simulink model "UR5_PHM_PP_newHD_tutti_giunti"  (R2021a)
settings: Solver=ode14x  StartTime=0.0  StopTime=Sim.time  FixedStep=Sim.dt  MaxStep=Sim.dt  RelTol=1e-3  EnableMultiTasking=on
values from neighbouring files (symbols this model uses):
  alpha_n = 0.98*pi/180    (= 0.0171042266695)    [parameters.m]
  alpha_t = 30*pi/180    (= 0.523598775598)    [parameters.m]
  alpha_TTS = 0    [parameters.m]
  alpha_Tw_L = -6.9e-4    (= -0.00069)    [parameters.m]
  alpha_Tw_R = 3.9e-3    (= 0.0039)    [parameters.m]
  Beta_TTS = 0    [parameters.m]
  c1 = 1e-2    (= 0.01)    [parameters.m]
  c2 = 1e-2    (= 0.01)    [parameters.m]
  c3 = 1e-2    (= 0.01)    [parameters.m]
  c4 = 1e-2    (= 0.01)    [parameters.m]
  c5 = 1e-2    (= 0.01)    [parameters.m]
  c6 = 1e-2    (= 0.01)    [parameters.m]
  Cb1 = 1.8e3    (= 1800)    [parameters.m]
  Cb2 = 1.8e3    (= 1800)    [parameters.m]
  Cb3 = 1.8e3    (= 1800)    [parameters.m]
  Cb4 = 1.8e3    (= 1800)    [parameters.m]
  Cb5 = 1.8e3    (= 1800)    [parameters.m]
  Cb6 = 1.8e3    (= 1800)    [parameters.m]
  Cth_housing = 153.90    (= 153.9)    [parameters.m]
  Cth_w = 74.20    (= 74.2)    [parameters.m]
  dt_PP = 0.05    [parameters.m]
  Fric1 = [fc_1/2 1e1 fc_1 fv_1]    [parameters.m]
  Fric2 = [fc_2/2 1e1 fc_2 fv_2]    [parameters.m]
  Fric3 = [fc_3/2 1e1 fc_3 fv_3]    [parameters.m]
  Fric4 = [fc_4/2 1e1 fc_4 fv_4]    [parameters.m]
  Fric5 = [fc_5/2 1e1 fc_5 fv_5]    [parameters.m]
  Fric6 = [fc_6/2 1e1 fc_6 fv_6]    [parameters.m]
  Hth_housing = 0.30    (= 0.3)    [parameters.m]
  Hth_w = 1.14    [parameters.m]
  I_actual = I_actual(1:10,:)    [trajcutting.m]
  J_CS1 = 7.12e-5    (= 7.12e-05)    [parameters.m]
  J_CS2 = 7.12e-5    (= 7.12e-05)    [parameters.m]
  J_CS3 = 7.12e-5    (= 7.12e-05)    [parameters.m]
  J_CS4 = 6e-6    (= 6e-06)    [parameters.m]
  J_CS5 = 6e-6    (= 6e-06)    [parameters.m]
  J_CS6 = 6e-6    (= 6e-06)    [parameters.m]
  J_FS1 = 1.62e-7    (= 1.62e-07)    [parameters.m]
  J_FS2 = 1.62e-7    (= 1.62e-07)    [parameters.m]
  J_FS3 = 1.62e-7    (= 1.62e-07)    [parameters.m]
  J_FS4 = 4.97e-8    (= 4.97e-08)    [parameters.m]
  J_FS5 = 4.97e-8    (= 4.97e-08)    [parameters.m]
  J_FS6 = 4.97e-8    (= 4.97e-08)    [parameters.m]
  J_WG1 = 3.56e-5    (= 3.56e-05)    [parameters.m]
  J_WG2 = 3.56e-5    (= 3.56e-05)    [parameters.m]
  J_WG3 = 3.56e-5    (= 3.56e-05)    [parameters.m]
  J_WG4 = 3e-6    (= 3e-06)    [parameters.m]
  J_WG5 = 3e-6    (= 3e-06)    [parameters.m]
  J_WG6 = 3e-6    (= 3e-06)    [parameters.m]
  K_i = 1    [parameters.m]
  K_p = 1    [parameters.m]
  K_torsCS1 = 4.78e6    (= 4780000)    [parameters.m]
  K_torsCS2 = 4.78e6    (= 4780000)    [parameters.m]
  K_torsCS3 = 4.78e6    (= 4780000)    [parameters.m]
  K_torsCS4 = 1.06e6    (= 1060000)    [parameters.m]
  K_torsCS5 = 1.06e6    (= 1060000)    [parameters.m]
  K_torsCS6 = 1.06e6    (= 1060000)    [parameters.m]
  K_torsWG1 = 9.56e5    (= 956000)    [parameters.m]
  K_torsWG2 = 9.56e5    (= 956000)    [parameters.m]
  K_torsWG3 = 9.56e5    (= 956000)    [parameters.m]
  K_torsWG4 = 1.84e5    (= 184000)    [parameters.m]
  K_torsWG5 = 1.84e5    (= 184000)    [parameters.m]
  K_torsWG6 = 1.84e5    (= 184000)    [parameters.m]
  K_v = 1    [parameters.m]
  Kb1 = 0.51e8    (= 51000000)    [parameters.m]
  Kb2 = 0.51e8    (= 51000000)    [parameters.m]
  Kb3 = 0.51e8    (= 51000000)    [parameters.m]
  Kb4 = 1.98e7    (= 19800000)    [parameters.m]
  Kb5 = 1.98e7    (= 19800000)    [parameters.m]
  Kb6 = 1.98e7    (= 19800000)    [parameters.m]
  Km1 = 1.2e9    (= 1200000000)    [parameters.m]
  Km2 = 1.2e9    (= 1200000000)    [parameters.m]
  Km3 = 1.2e9    (= 1200000000)    [parameters.m]
  Km4 = 5.55e8    (= 555000000)    [parameters.m]
  Km5 = 5.55e8    (= 555000000)    [parameters.m]
  Km6 = 5.55e8    (= 555000000)    [parameters.m]
  Kt1 = 0.96e5    (= 96000)    [parameters.m]
  Kt2 = 0.96e5    (= 96000)    [parameters.m]
  Kt3 = 0.96e5    (= 96000)    [parameters.m]
  Kt4 = 1.15e4    (= 11500)    [parameters.m]
  Kt5 = 1.15e4    (= 11500)    [parameters.m]
  Kt6 = 1.15e4    (= 11500)    [parameters.m]
  L = Motor.L_2/2    [parameters.m]
  m2 = polyfit(Temp(:,2),pBn_UR5_f_Temp(:,2),1)    [parameters.m]
  mb2 = polyfit(Temp(:,8),pBn_UR5_f_Temp(:,8),1)    [parameters.m]
  pickTime = t_pick(traj)    [parameters.m]
  placeTime = t_place(traj)    [parameters.m]
  q0 = q_target(1,:)    [testlaw_PP.m]
  q_CS01 = x(6)    [parameters.m]
  q_CS02 = x(6)    [parameters.m]
  q_CS03 = x(6)    [parameters.m]
  q_CS04 = x(6)    [parameters.m]
  q_CS05 = x(6)    [parameters.m]
  q_CS06 = x(6)    [parameters.m]
  q_WG01 = x(1)    [parameters.m]
  q_WG02 = x(1)    [parameters.m]
  q_WG03 = x(1)    [parameters.m]
  q_WG04 = x(1)    [parameters.m]
  q_WG05 = x(1)    [parameters.m]
  q_WG06 = x(1)    [parameters.m]
  quant_i = [Motor.imax1 Motor.imax2      Motor.imax3 Motor.imax4 Motor.imax5 Motor.imax6]/2^16    [parameters.m]
  R = Motor.R_2/2    [parameters.m]
  rg1 = 0.028    [parameters.m]
  rg2 = 0.028    [parameters.m]
  rg3 = 0.028    [parameters.m]
  rg4 = 0.0155    [parameters.m]
  rg5 = 0.0155    [parameters.m]
  rg6 = 0.0155    [parameters.m]
  sigma_p = 444.29    [parameters.m]
  sigma_v = 2*pi*1000    (= 6283.18530718)    [parameters.m]
  stiff_red = 1    [parameters.m]
  T_0 = Sim.temp    [parameters.m]
  T_switch = 1e-4    (= 0.0001)    [parameters.m]
  tau_i = 1/(fc_i*2*pi)    (= 7.95774715459e-05)    [parameters.m]
  U_s = 48    [parameters.m]
  var_i = 1e-1*[.0167 .0184 .0144 .0016      .0011 .0007]    [parameters.m]
  var_p = 1e-6*[.0943 .3877      .3478 .5436 .3400 .2081]    [parameters.m]
  var_v = 1e-4*[.0738 .1452      .1564 .4623 .1824 .0917]    [parameters.m]
  Wf_TTS_0 = 0    [parameters.m]
  Wf_TTS_ONOFF = 0    [parameters.m]
  x2_01 = x(3)    [parameters.m]
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undefined symbols (not defined in the file or in its folder): deg, Driver1, Driver2, Driver3, Driver4, Driver5, Driver6, elseif, geom, Ground, J1, J2, J3, J4, J5, J6, kg, L1, L2, L3, L4, L5, L6, LINK0, LINK1, LINK2, LINK3, LINK4, LINK5, LINK6, m, Motor, N, payload, ROBOTIQ_FT, s, Sim, Tool, X, Y, Z
libraries: sm_lib x35, nesl_utility x30, simulink x23, simulink_extras x11, spsTriangleGeneratorLib x6
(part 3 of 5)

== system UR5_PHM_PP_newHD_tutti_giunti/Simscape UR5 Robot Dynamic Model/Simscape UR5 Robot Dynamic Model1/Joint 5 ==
  T5 : Inport
  A_45*E_1 : sm_lib/Frames and Transforms/Rigid Transform  TranslationMethod=Cartesian  TranslationStandardOffset=0  TranslationLengthUnit=mm  TranslationStandardAxis=+Z  TranslationCartesianOffset=A45t  TranslationROffset=0  TranslationROffsetUnits=m  TranslationZOffset=0  TranslationZOffsetUnits=m  TranslationThetaOffset=0  TranslationThetaOffsetUnits=deg  RotationMethod=None  RotationAngleUnits=deg  RotationStandardAxis=+Z  RotationAngle=0.0  RotationArbitraryAxis=[0 0 1]  FollAlignAxisA=+X  BaseAlignAxisA=+Y  FollAlignAxisB=+Y  BaseAlignAxisB=+Z  RotationSequenceAxes=FollowerAxes  RotationSequence=XYX  RotationSequenceAngles=[0 0 0]  RotationSequenceAnglesUnits=deg  RotationMatrix=A45r
  A_45*E_45 : sm_lib/Frames and Transforms/Rigid Transform  TranslationMethod=None  TranslationStandardOffset=0  TranslationLengthUnit=mm  TranslationStandardAxis=+Z  TranslationCartesianOffset=A45t  TranslationROffset=0  TranslationROffsetUnits=m  TranslationZOffset=0  TranslationZOffsetUnits=m  TranslationThetaOffset=0  TranslationThetaOffsetUnits=deg  RotationMethod=RotationMatrix  RotationAngleUnits=deg  RotationStandardAxis=+Z  RotationAngle=0.0  RotationArbitraryAxis=[0 0 1]  FollAlignAxisA=+X  BaseAlignAxisA=+Y  FollAlignAxisB=+Y  BaseAlignAxisB=+Z  RotationSequenceAxes=FollowerAxes  RotationSequence=XYX  RotationSequenceAngles=[0 0 0]  RotationSequenceAnglesUnits=deg  RotationMatrix=A45r
  Mux : Mux  Inputs=3
  PS-Simulink Converter1 : nesl_utility/PS-Simulink Converter  PhysicalDomain=network_engine_domain  SubClassName=ps_output  LeftPortType=input  RightPortType=output  PseudoPeriodic=off  Frequencies=[]  Unit=1  AffineConversion=off
  PS-Simulink Converter2 : nesl_utility/PS-Simulink Converter  PhysicalDomain=network_engine_domain  SubClassName=ps_output  LeftPortType=input  RightPortType=output  PseudoPeriodic=off  Frequencies=[]  Unit=1  AffineConversion=off
  PS-Simulink Converter7 : nesl_utility/PS-Simulink Converter  PhysicalDomain=network_engine_domain  SubClassName=ps_output  LeftPortType=input  RightPortType=output  PseudoPeriodic=off  Frequencies=[]  Unit=1  AffineConversion=off
  Revolute Joint5 : sm_lib/Joints/Revolute Joint  JointMode=Normal  SenseConstraintForce=off  SenseConstraintForceX=off  SenseConstraintForceY=off  SenseConstraintForceZ=off  SenseConstraintTorque=off  SenseConstraintTorqueX=off  SenseConstraintTorqueY=off  SenseConstraintTorqueZ=off  SenseTotalForce=off  SenseTotalForceX=off  SenseTotalForceY=off  SenseTotalForceZ=off  SenseTotalTorque=off  SenseTotalTorqueX=off  SenseTotalTorqueY=off  SenseTotalTorqueZ=off  CompositeWrenchDir=FollowerOnBase  CompositeWrenchFrame=BaseFrame  EquilibriumPosition=0  EquilibriumPositionUnits=deg  SpringStiffness=0  SpringStiffnessUnits=N*m/deg  DampingCoefficient=0  DampingCoefficientUnits=N*m/(deg/s)  TorqueActuationMode=InputTorque  MotionActuationMode=ComputedMotion  SensePosition=on  SenseVelocity=on  SenseAcceleration=on  SenseTorqueForce=off  SenseLowerLimitTorqueForce=off  SenseUpperLimitTorqueForce=off  LowerLimitSpecify=on  LowerLimitBound=-J5.al  LowerLimitBoundUnits=deg  LowerLimitStiffness=1e4  LowerLimitStiffnessUnits=N*m/deg  LowerLimitDamping=10  LowerLimitDampingUnits=N*m/(deg/s)  LowerLimitTransitionRegionWidth=0.1  LowerLimitTransitionRegionWidthUnits=deg  UpperLimitSpecify=on  UpperLimitBound=J5.al  UpperLimitBoundUnits=deg  UpperLimitStiffness=1e4  UpperLimitStiffnessUnits=N*m/deg  UpperLimitDamping=10  UpperLimitDampingUnits=N*m/(deg/s)  UpperLimitTransitionRegionWidth=0.1  UpperLimitTransitionRegionWidthUnits=deg  PositionTargetSpecify=on  PositionTargetPriority=Low  PositionTargetValue=q0(5)  PositionTargetValueUnits=rad  VelocityTargetSpecify=off  VelocityTargetPriority=High  VelocityTargetValue=0  VelocityTargetValueUnits=deg/s
  Simulink-PS Converter : nesl_utility/Simulink-PS Converter  PhysicalDomain=network_engine_domain  SubClassName=ps_input  LeftPortType=input  RightPortType=output  PseudoPeriodic=off  Frequencies=[]  NoiseDistribution=none  NoiseParameters=[]  Unit=1  AffineConversion=off  FilteringAndDerivatives=provide  SimscapeFilterOrder=1  InputFilterTimeConstant=0.001  UdotUserProvided=0
  Link 4 : PMIOPort  Side=Left
  Link 5 : PMIOPort  Port=2  Side=Right
  q5,qd5,qdd5 : Outport
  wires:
  PS-Simulink Converter1/1 -> Mux/1
  T5/1 -> Simulink-PS Converter/1
  Mux/1 -> q5,qd5,qdd5/1
  PS-Simulink Converter7/1 -> Mux/2
  PS-Simulink Converter2/1 -> Mux/3
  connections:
  A_45*E_45/RConn1 -- A_45*E_1/LConn1
  A_45*E_1/RConn1 -- Revolute Joint5/LConn1
  A_45*E_45/LConn1 -- Link 4/RConn1
  Revolute Joint5/RConn1 -- Link 5/RConn1
  Revolute Joint5/RConn4 -- PS-Simulink Converter2/LConn1
  Revolute Joint5/LConn2 -- Simulink-PS Converter/RConn1
  Revolute Joint5/RConn3 -- PS-Simulink Converter7/LConn1
  Revolute Joint5/RConn2 -- PS-Simulink Converter1/LConn1

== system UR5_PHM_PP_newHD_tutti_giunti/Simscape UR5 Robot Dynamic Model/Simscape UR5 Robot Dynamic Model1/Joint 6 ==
  T6 : Inport
  A_56*E_1 : sm_lib/Frames and Transforms/Rigid Transform  TranslationMethod=Cartesian  TranslationStandardOffset=0  TranslationLengthUnit=mm  TranslationStandardAxis=+Z  TranslationCartesianOffset=A56t  TranslationROffset=0  TranslationROffsetUnits=m  TranslationZOffset=0  TranslationZOffsetUnits=m  TranslationThetaOffset=0  TranslationThetaOffsetUnits=deg  RotationMethod=None  RotationAngleUnits=deg  RotationStandardAxis=+Z  RotationAngle=0.0  RotationArbitraryAxis=[0 0 1]  FollAlignAxisA=+X  BaseAlignAxisA=+Y  FollAlignAxisB=+Y  BaseAlignAxisB=+Z  RotationSequenceAxes=FollowerAxes  RotationSequence=XYX  RotationSequenceAngles=[0 0 0]  RotationSequenceAnglesUnits=deg  RotationMatrix=A56r
  A_56*E_56 : sm_lib/Frames and Transforms/Rigid Transform  TranslationMethod=None  TranslationStandardOffset=0  TranslationLengthUnit=mm  TranslationStandardAxis=+Z  TranslationCartesianOffset=A56t  TranslationROffset=0  TranslationROffsetUnits=m  TranslationZOffset=0  TranslationZOffsetUnits=m  TranslationThetaOffset=0  TranslationThetaOffsetUnits=deg  RotationMethod=RotationMatrix  RotationAngleUnits=deg  RotationStandardAxis=+Z  RotationAngle=0.0  RotationArbitraryAxis=[0 0 1]  FollAlignAxisA=+X  BaseAlignAxisA=+Y  FollAlignAxisB=+Y  BaseAlignAxisB=+Z  RotationSequenceAxes=FollowerAxes  RotationSequence=XYX  RotationSequenceAngles=[0 0 0]  RotationSequenceAnglesUnits=deg  RotationMatrix=A56r
  Mux : Mux  Inputs=3
  PS-Simulink Converter1 : nesl_utility/PS-Simulink Converter  PhysicalDomain=network_engine_domain  SubClassName=ps_output  LeftPortType=input  RightPortType=output  PseudoPeriodic=off  Frequencies=[]  Unit=1  AffineConversion=off
  PS-Simulink Converter2 : nesl_utility/PS-Simulink Converter  PhysicalDomain=network_engine_domain  SubClassName=ps_output  LeftPortType=input  RightPortType=output  PseudoPeriodic=off  Frequencies=[]  Unit=1  AffineConversion=off
  PS-Simulink Converter7 : nesl_utility/PS-Simulink Converter  PhysicalDomain=network_engine_domain  SubClassName=ps_output  LeftPortType=input  RightPortType=output  PseudoPeriodic=off  Frequencies=[]  Unit=1  AffineConversion=off
  Revolute Joint6 : sm_lib/Joints/Revolute Joint  JointMode=Normal  SenseConstraintForce=off  SenseConstraintForceX=off  SenseConstraintForceY=off  SenseConstraintForceZ=off  SenseConstraintTorque=off  SenseConstraintTorqueX=off  SenseConstraintTorqueY=off  SenseConstraintTorqueZ=off  SenseTotalForce=off  SenseTotalForceX=off  SenseTotalForceY=off  SenseTotalForceZ=off  SenseTotalTorque=off  SenseTotalTorqueX=off  SenseTotalTorqueY=off  SenseTotalTorqueZ=off  CompositeWrenchDir=FollowerOnBase  CompositeWrenchFrame=BaseFrame  EquilibriumPosition=0  EquilibriumPositionUnits=deg  SpringStiffness=0  SpringStiffnessUnits=N*m/deg  DampingCoefficient=0  DampingCoefficientUnits=N*m/(deg/s)  TorqueActuationMode=InputTorque  MotionActuationMode=ComputedMotion  SensePosition=on  SenseVelocity=on  SenseAcceleration=on  SenseTorqueForce=off  SenseLowerLimitTorqueForce=off  SenseUpperLimitTorqueForce=off  LowerLimitSpecify=on  LowerLimitBound=-J6.al  LowerLimitBoundUnits=deg  LowerLimitStiffness=1e4  LowerLimitStiffnessUnits=N*m/deg  LowerLimitDamping=10  LowerLimitDampingUnits=N*m/(deg/s)  LowerLimitTransitionRegionWidth=0.1  LowerLimitTransitionRegionWidthUnits=deg  UpperLimitSpecify=on  UpperLimitBound=J6.al  UpperLimitBoundUnits=deg  UpperLimitStiffness=1e4  UpperLimitStiffnessUnits=N*m/deg  UpperLimitDamping=10  UpperLimitDampingUnits=N*m/(deg/s)  UpperLimitTransitionRegionWidth=0.1  UpperLimitTransitionRegionWidthUnits=deg  PositionTargetSpecify=on  PositionTargetPriority=Low  PositionTargetValue=q0(6)  PositionTargetValueUnits=rad  VelocityTargetSpecify=off  VelocityTargetPriority=High  VelocityTargetValue=0  VelocityTargetValueUnits=deg/s
  Simulink-PS Converter : nesl_utility/Simulink-PS Converter  PhysicalDomain=network_engine_domain  SubClassName=ps_input  LeftPortType=input  RightPortType=output  PseudoPeriodic=off  Frequencies=[]  NoiseDistribution=none  NoiseParameters=[]  Unit=1  AffineConversion=off  FilteringAndDerivatives=provide  SimscapeFilterOrder=1  InputFilterTimeConstant=0.001  UdotUserProvided=0
  Link 5 : PMIOPort  Side=Left
  Link 6 : PMIOPort  Port=2  Side=Right
  q6,qd6,qdd6 : Outport
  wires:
  PS-Simulink Converter1/1 -> Mux/1
  T6/1 -> Simulink-PS Converter/1
  Mux/1 -> q6,qd6,qdd6/1
  PS-Simulink Converter7/1 -> Mux/2
  PS-Simulink Converter2/1 -> Mux/3
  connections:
  A_56*E_1/LConn1 -- A_56*E_56/RConn1
  Revolute Joint6/LConn1 -- A_56*E_1/RConn1
  Revolute Joint6/RConn1 -- Link 6/RConn1
  A_56*E_56/LConn1 -- Link 5/RConn1
  Revolute Joint6/RConn4 -- PS-Simulink Converter2/LConn1
  Revolute Joint6/LConn2 -- Simulink-PS Converter/RConn1
  Revolute Joint6/RConn3 -- PS-Simulink Converter7/LConn1
  Revolute Joint6/RConn2 -- PS-Simulink Converter1/LConn1

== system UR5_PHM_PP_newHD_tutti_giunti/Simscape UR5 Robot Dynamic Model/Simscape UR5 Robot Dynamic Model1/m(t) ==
  Add : Sum  Inputs=++++
  Ramp : simulink/Sources/Ramp  slope=payload.m/dt_PP  start=pickTime  InitialOutput=0.001
  Ramp1 : simulink/Sources/Ramp  slope=-payload.m/dt_PP  start=pickTime+dt_PP  InitialOutput=0.001
  Ramp2 : simulink/Sources/Ramp  slope=-payload.m/dt_PP  start=placeTime  InitialOutput=0.001
  Ramp3 : simulink/Sources/Ramp  slope=payload.m/dt_PP  start=placeTime+dt_PP  InitialOutput=0.001
  Out1 : Outport
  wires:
  Ramp2/1 -> Add/3
  Ramp/1 -> Add/1
  Ramp3/1 -> Add/4
  Ramp1/1 -> Add/2
  Add/1 -> Out1/1

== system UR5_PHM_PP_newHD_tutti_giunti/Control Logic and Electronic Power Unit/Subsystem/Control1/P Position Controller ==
  q_error : Inport
  "[-pi*tau,pi*tau]" : Saturate  UpperLimit=pi*Motor.tau  LowerLimit=-pi*Motor.tau
  kp_p : Gain  Gain=Driver1.Pp
  qdm_ref : Outport
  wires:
  kp_p/1 -> "[-pi*tau,pi*tau]"/1
  q_error/1 -> kp_p/1
  "[-pi*tau,pi*tau]"/1 -> qdm_ref/1

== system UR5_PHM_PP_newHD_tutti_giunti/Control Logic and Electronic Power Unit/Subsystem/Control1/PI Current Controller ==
  i_error : Inport
  Integral Contribution : Scope
  Integrator : Integrator
  Proportional Contribution : Scope
  Sum3 : Sum  Inputs=|++
  "[-U_s,U_s]" : Saturate  UpperLimit=U_s  LowerLimit=-U_s
  ki_i : Gain  Gain=Driver1.Ii
  kp_i : Gain  Gain=Driver1.Pi
  V_ref : Outport
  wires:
  i_error/1 -> ki_i/1, kp_i/1
  kp_i/1 -> Sum3/1, Proportional Contribution/1
  "[-U_s,U_s]"/1 -> V_ref/1
  Sum3/1 -> "[-U_s,U_s]"/1
  ki_i/1 -> Integrator/1
  Integrator/1 -> Integral Contribution/1, Sum3/2

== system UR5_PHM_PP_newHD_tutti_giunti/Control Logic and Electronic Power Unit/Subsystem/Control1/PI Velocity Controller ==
  qdm_error : Inport
  Current : Scope
  Integral Contribution : Scope
  Integrator : Integrator
  Proportional Contribution : Scope
  Sum3 : Sum  Inputs=|++
  "[-i_max,i_max]" : Saturate  UpperLimit=Motor.imax1  LowerLimit=-Motor.imax1
  ki_v : Gain  Gain=Driver1.Iv
  kp_v : Gain  Gain=Driver1.Pv
  i_ref : Outport
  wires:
  Sum3/1 -> "[-i_max,i_max]"/1
  "[-i_max,i_max]"/1 -> Current/1, i_ref/1
  kp_v/1 -> Proportional Contribution/1, Sum3/1
  qdm_error/1 -> ki_v/1, kp_v/1
  ki_v/1 -> Integrator/1
  Integrator/1 -> Sum3/2, Integral Contribution/1

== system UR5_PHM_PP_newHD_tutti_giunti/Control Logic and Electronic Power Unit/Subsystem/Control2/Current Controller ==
  i_ref : Inport
  i_FB [dq0] : Inport  Port=2
  Controller - d : Subsystem
  Controller - q : Subsystem
  Demux : Demux  Outputs=3
  Mux : Mux  Inputs=3
  V[d,q,0] : Outport
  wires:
  Controller - d/1(v*d) -> Mux/1  "vd_j2"
  Demux/3 -> Mux/3  "i0_j2"
  Controller - q/1(v*q) -> Mux/2  "vq_j2"
  Demux/2 -> Controller - q/2(Iq)  "iq_j2"
  i_ref/1 -> Controller - q/1(i*)
  i_FB [dq0]/1 -> Demux/1
  Demux/1 -> Controller - d/1(id)  "id_j2"
  Mux/1 -> V[d,q,0]/1

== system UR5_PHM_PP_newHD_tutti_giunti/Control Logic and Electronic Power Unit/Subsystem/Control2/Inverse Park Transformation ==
  V[d,q,0] : Inport
  qm : Inport  Port=2
  A11 : Fcn  Expr=sin(u(1))
  A12 : Fcn  Expr=cos(u(1))
  A13 : Fcn  Expr=sqrt(2)/2
  A21 : Fcn  Expr=sin(u(1)-2/3*pi)
  A22 : Fcn  Expr=cos(u(1)-2/3*pi)
  A23 : Fcn  Expr=sqrt(2)/2
  A31 : Fcn  Expr=sin(u(1)+2/3*pi)
  A32 : Fcn  Expr=cos(u(1)+2/3*pi)
  A33 : Fcn  Expr=sqrt(2)/2
  Gain : Gain  Gain=sqrt(2/3)
  Gain1 : Gain  Gain=Motor.Zp_2
  Matrix : Subsystem
  Product : Product  Multiplication=Matrix(*)  RndMeth=Zero
  V[a,b,c] : Outport  VectorParamsAs1DForOutWhenUnconnected=off
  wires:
  Product/1 -> V[a,b,c]/1
  V[d,q,0]/1 -> Product/2
  Gain/1 -> Product/1
  Gain1/1 -> A22/1, A21/1, A11/1, A12/1, A13/1, A31/1, A32/1, A33/1, A23/1
  A11/1 -> Matrix/1(A11)
  A23/1 -> Matrix/6(A23)
  A12/1 -> Matrix/2(A12)
  A21/1 -> Matrix/4(A21)
  qm/1 -> Gain1/1
  A33/1 -> Matrix/9(A33)
  Matrix/1(Out1) -> Gain/1
  A13/1 -> Matrix/3(A13)
  A22/1 -> Matrix/5(A22)
  A32/1 -> Matrix/8(A32)
  A31/1 -> Matrix/7(A31)

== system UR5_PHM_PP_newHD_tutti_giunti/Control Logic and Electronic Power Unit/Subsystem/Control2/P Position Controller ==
  q_error : Inport
  "[-pi*tau,pi*tau]" : Saturate  UpperLimit=pi*Motor.tau  LowerLimit=-pi*Motor.tau
  kp_p : Gain  Gain=Driver2.Pp
  qdm_ref : Outport
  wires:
  q_error/1 -> kp_p/1
  "[-pi*tau,pi*tau]"/1 -> qdm_ref/1
  kp_p/1 -> "[-pi*tau,pi*tau]"/1

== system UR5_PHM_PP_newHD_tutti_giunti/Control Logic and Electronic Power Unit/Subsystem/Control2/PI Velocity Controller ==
  qdm_error : Inport
  Add : Sum
  Integral Contribution : Scope
  Integrator1 : Integrator
  Proportional Contribution : Scope
  Scope i_ref : Scope  NumInputPorts=2
  "[-i_max,i_max]" : Saturate  UpperLimit=Motor.imax2  LowerLimit=-Motor.imax2
  ki_v : Gain  Gain=Driver2.Iv
  kp_v : Gain  Gain=Driver2.Pv
  i_ref : Outport
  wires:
  Integrator1/1 -> Integral Contribution/1, Add/2
  qdm_error/1 -> ki_v/1, kp_v/1
  kp_v/1 -> Proportional Contribution/1, Add/1
  Add/1 -> Scope i_ref/1, "[-i_max,i_max]"/1
  "[-i_max,i_max]"/1 -> i_ref/1, Scope i_ref/2
  ki_v/1 -> Integrator1/1

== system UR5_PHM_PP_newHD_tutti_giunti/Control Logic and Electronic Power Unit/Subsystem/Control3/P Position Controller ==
  q_error : Inport
  "[-pi*tau,pi*tau]" : Saturate  UpperLimit=pi*Motor.tau  LowerLimit=-pi*Motor.tau
  kp_p : Gain  Gain=Driver2.Pp
  qdm_ref : Outport
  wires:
  kp_p/1 -> "[-pi*tau,pi*tau]"/1
  q_error/1 -> kp_p/1
  "[-pi*tau,pi*tau]"/1 -> qdm_ref/1

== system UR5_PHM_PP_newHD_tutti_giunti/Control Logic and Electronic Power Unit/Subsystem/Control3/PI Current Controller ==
  i_error : Inport
  Integral Contribution : Scope
  Integrator : Integrator
  Proportional Contribution : Scope
  Sum3 : Sum  Inputs=|++
  "[-U_s,U_s]" : Saturate  UpperLimit=U_s  LowerLimit=-U_s
  ki_i : Gain  Gain=Driver3.Ii
  kp_i : Gain  Gain=Driver3.Pi
  V_ref : Outport
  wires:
  i_error/1 -> ki_i/1, kp_i/1
  kp_i/1 -> Sum3/1, Proportional Contribution/1
  "[-U_s,U_s]"/1 -> V_ref/1
  Sum3/1 -> "[-U_s,U_s]"/1
  Integrator/1 -> Sum3/2, Integral Contribution/1
  ki_i/1 -> Integrator/1

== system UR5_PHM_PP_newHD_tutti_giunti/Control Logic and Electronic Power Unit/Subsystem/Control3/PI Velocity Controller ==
  qdm_error : Inport
  Integral Contribution : Scope
  Integrator : Integrator
  Proportional Contribution : Scope
  Sum3 : Sum  Inputs=|++
  "[-i_max,i_max]" : Saturate  UpperLimit=Motor.imax3  LowerLimit=-Motor.imax3
  ki_v : Gain  Gain=Driver3.Iv
  kp_v : Gain  Gain=Driver3.Pv
  i_ref : Outport
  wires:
  Sum3/1 -> "[-i_max,i_max]"/1
  "[-i_max,i_max]"/1 -> i_ref/1
  kp_v/1 -> Proportional Contribution/1, Sum3/1
  qdm_error/1 -> ki_v/1, kp_v/1
  ki_v/1 -> Integrator/1
  Integrator/1 -> Sum3/2, Integral Contribution/1

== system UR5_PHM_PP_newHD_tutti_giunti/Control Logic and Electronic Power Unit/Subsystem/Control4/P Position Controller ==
  q_error : Inport
  "[-pi*tau,pi*tau]" : Saturate  UpperLimit=pi*Motor.tau  LowerLimit=-pi*Motor.tau
  kp_p : Gain  Gain=Driver4.Pp
  qdm_ref : Outport
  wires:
  kp_p/1 -> "[-pi*tau,pi*tau]"/1
  q_error/1 -> kp_p/1
  "[-pi*tau,pi*tau]"/1 -> qdm_ref/1

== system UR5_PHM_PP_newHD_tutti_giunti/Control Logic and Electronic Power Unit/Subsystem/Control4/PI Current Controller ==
  i_error : Inport
  Integral Contribution : Scope
  Integrator : Integrator
  Proportional Contribution : Scope
  Sum3 : Sum  Inputs=|++
  "[-U_s,U_s]" : Saturate  UpperLimit=U_s  LowerLimit=-U_s
  ki_i : Gain  Gain=Driver4.Ii
  kp_i : Gain  Gain=Driver4.Pi
  V_ref : Outport
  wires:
  i_error/1 -> ki_i/1, kp_i/1
  kp_i/1 -> Sum3/1, Proportional Contribution/1
  "[-U_s,U_s]"/1 -> V_ref/1
  Sum3/1 -> "[-U_s,U_s]"/1
  ki_i/1 -> Integrator/1
  Integrator/1 -> Sum3/2, Integral Contribution/1

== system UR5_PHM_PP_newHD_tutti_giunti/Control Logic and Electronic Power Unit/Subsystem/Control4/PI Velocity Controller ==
  qdm_error : Inport
  Integral Contribution : Scope
  Integrator : Integrator
  Proportional Contribution : Scope
  Sum3 : Sum  Inputs=|++
  "[-i_max,i_max]" : Saturate  UpperLimit=Motor.imax4  LowerLimit=-Motor.imax4
  ki_v : Gain  Gain=Driver4.Iv
  kp_v : Gain  Gain=Driver4.Pv
  i_ref : Outport
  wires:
  Sum3/1 -> "[-i_max,i_max]"/1
  "[-i_max,i_max]"/1 -> i_ref/1
  kp_v/1 -> Proportional Contribution/1, Sum3/1
  qdm_error/1 -> ki_v/1, kp_v/1
  ki_v/1 -> Integrator/1
  Integrator/1 -> Sum3/2, Integral Contribution/1

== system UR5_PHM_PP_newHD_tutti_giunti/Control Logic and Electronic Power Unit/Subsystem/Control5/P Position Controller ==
  q_error : Inport
  "[-pi*tau,pi*tau]" : Saturate  UpperLimit=pi*Motor.tau  LowerLimit=-pi*Motor.tau
  kp_p : Gain  Gain=Driver5.Pp
  qdm_ref : Outport
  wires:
  kp_p/1 -> "[-pi*tau,pi*tau]"/1
  q_error/1 -> kp_p/1
  "[-pi*tau,pi*tau]"/1 -> qdm_ref/1

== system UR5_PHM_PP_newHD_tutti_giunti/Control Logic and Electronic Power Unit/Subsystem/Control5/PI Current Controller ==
  i_error : Inport
  Integral Contribution : Scope
  Integrator : Integrator
  Proportional Contribution : Scope
  Sum3 : Sum  Inputs=|++
  "[-U_s,U_s]" : Saturate  UpperLimit=U_s  LowerLimit=-U_s
  ki_i : Gain  Gain=Driver5.Ii
  kp_i : Gain  Gain=Driver5.Pi
  V_ref : Outport
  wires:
  i_error/1 -> ki_i/1, kp_i/1
  kp_i/1 -> Sum3/1, Proportional Contribution/1
  "[-U_s,U_s]"/1 -> V_ref/1
  Sum3/1 -> "[-U_s,U_s]"/1
  ki_i/1 -> Integrator/1
  Integrator/1 -> Integral Contribution/1, Sum3/2

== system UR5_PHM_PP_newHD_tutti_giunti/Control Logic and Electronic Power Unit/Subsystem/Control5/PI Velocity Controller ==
  qdm_error : Inport
  Integral Contribution : Scope
  Integrator : Integrator
  Proportional Contribution : Scope
  Sum3 : Sum  Inputs=|++
  "[-i_max,i_max]" : Saturate  UpperLimit=Motor.imax5  LowerLimit=-Motor.imax5
  ki_v : Gain  Gain=Driver5.Iv
  kp_v : Gain  Gain=Driver5.Pv
  i_ref : Outport
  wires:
  Sum3/1 -> "[-i_max,i_max]"/1
  "[-i_max,i_max]"/1 -> i_ref/1
  kp_v/1 -> Proportional Contribution/1, Sum3/1
  qdm_error/1 -> ki_v/1, kp_v/1
  ki_v/1 -> Integrator/1
  Integrator/1 -> Sum3/2, Integral Contribution/1

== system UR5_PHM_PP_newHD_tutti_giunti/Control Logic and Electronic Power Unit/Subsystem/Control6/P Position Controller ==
  q_error : Inport
  "[-pi*tau,pi*tau]" : Saturate  UpperLimit=pi*Motor.tau  LowerLimit=-pi*Motor.tau
  kp_p : Gain  Gain=Driver6.Pp
  qdm_ref : Outport
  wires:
  kp_p/1 -> "[-pi*tau,pi*tau]"/1
  q_error/1 -> kp_p/1
  "[-pi*tau,pi*tau]"/1 -> qdm_ref/1

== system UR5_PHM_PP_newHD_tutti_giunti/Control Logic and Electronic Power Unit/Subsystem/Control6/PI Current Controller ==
  i_error : Inport
  Integral Contribution : Scope
  Integrator : Integrator
  Proportional Contribution : Scope
  Sum3 : Sum  Inputs=|++
  "[-U_s,U_s]" : Saturate  UpperLimit=U_s  LowerLimit=-U_s
  ki_i : Gain  Gain=Driver6.Ii
  kp_i : Gain  Gain=Driver6.Pi
  V_ref : Outport
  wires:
  i_error/1 -> ki_i/1, kp_i/1
  kp_i/1 -> Sum3/1, Proportional Contribution/1
  "[-U_s,U_s]"/1 -> V_ref/1
  Sum3/1 -> "[-U_s,U_s]"/1
  ki_i/1 -> Integrator/1
  Integrator/1 -> Sum3/2, Integral Contribution/1

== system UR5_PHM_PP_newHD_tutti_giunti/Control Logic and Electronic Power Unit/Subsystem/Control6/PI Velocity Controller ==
  qdm_error : Inport
  Integral Contribution : Scope
  Integrator : Integrator
  Proportional Contribution : Scope
  Sum3 : Sum  Inputs=|++
  "[-i_max,i_max]" : Saturate  UpperLimit=Motor.imax6  LowerLimit=-Motor.imax6
  ki_v : Gain  Gain=Driver6.Iv
  kp_v : Gain  Gain=Driver6.Pv
  i_ref : Outport
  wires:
  Sum3/1 -> "[-i_max,i_max]"/1
  "[-i_max,i_max]"/1 -> i_ref/1
  kp_v/1 -> Proportional Contribution/1, Sum3/1
  qdm_error/1 -> ki_v/1, kp_v/1
  ki_v/1 -> Integrator/1
  Integrator/1 -> Sum3/2, Integral Contribution/1

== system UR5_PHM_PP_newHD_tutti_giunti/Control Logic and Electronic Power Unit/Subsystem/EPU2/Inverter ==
  q[a,b,c] : Inport
  V_dclink : Inport  Port=2
  Add : Sum  Inputs=+-
  Add1 : Sum  Inputs=-+
  Constant : Constant  Value=[1;1;1]
  Constant1 : Constant  Value=[1;1;1]
  Gain : Gain  Gain=1/2
  Gain2 : Gain  Gain=2
  Gain3 : Gain  Gain=1/3
  Product : Product
  Product1 : Product
  Sum of Elements : Sum  Inputs=+
  V[ao,bo,co] : Outport  VectorParamsAs1DForOutWhenUnconnected=off
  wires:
  Constant1/1 -> Product1/2
  Gain/1 -> Product/1
  Product/1 -> Add1/2, Sum of Elements/1
  Sum of Elements/1 -> Gain3/1
  Add1/1 -> V[ao,bo,co]/1
  Product1/1 -> Add1/1
  q[a,b,c]/1 -> Gain2/1
  Add/1 -> Product/2
  Gain3/1 -> Product1/1
  V_dclink/1 -> Gain/1
  Gain2/1 -> Add/1
  Constant/1 -> Add/2

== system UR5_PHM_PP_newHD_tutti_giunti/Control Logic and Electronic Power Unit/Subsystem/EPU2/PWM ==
  V*[a,b,c] : Inport
  V_dclink : Inport  Port=2
  Data Type Conversion : DataTypeConversion  OutDataTypeStr=double
  Data Type Conversion1 : DataTypeConversion  OutDataTypeStr=double
  Data Type Conversion2 : DataTypeConversion  OutDataTypeStr=double
  Demux : Demux  Outputs=3
  Divide : Product  Inputs=*/
  Divide1 : Product  Inputs=*/
  Divide2 : Product  Inputs=*/
  Gain : Gain  Gain=1/2
  Gain1 : Gain  Gain=1/2
  Gain2 : Gain  Gain=1/2
  Mux : Mux  Inputs=[1;1;1]
  Relational Operator : RelationalOperator  OutDataTypeStr=boolean
  Relational Operator1 : RelationalOperator  OutDataTypeStr=boolean
  Relational Operator2 : RelationalOperator  OutDataTypeStr=boolean
  Saturation : Saturate  UpperLimit=1.01  LowerLimit=-1.01
  Saturation1 : Saturate  UpperLimit=1.01  LowerLimit=-1.01
  Saturation2 : Saturate  UpperLimit=1.01  LowerLimit=-1.01
  Triangle Generator : spsTriangleGeneratorLib/Triangle Generator  Freq=1/T_switch  Phase=0  Ts=0
  portante triangolare bipolare unitaria : simulink/Sources/Repeating Sequence  Commented=on  rep_seq_t=[0 T_switch/2 T_switch]  rep_seq_y=[-1 1 -1]
  q[a,b,c] : Outport  VectorParamsAs1DForOutWhenUnconnected=off
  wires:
  Triangle Generator/1 -> [carrier]
  [carrier] -> Relational Operator/2
  V_dclink/1 -> [V_dclink]
  Relational Operator/1 -> Data Type Conversion/1
  V*[a,b,c]/1 -> Demux/1
  Demux/1 -> Divide/1
  [V_dclink] -> Gain/1
  Gain/1 -> Divide/2
  Demux/2 -> Divide1/1
  [V_dclink] -> Gain1/1
  Gain1/1 -> Divide1/2
  Demux/3 -> Divide2/1
  [V_dclink] -> Gain2/1
  Gain2/1 -> Divide2/2
  Divide/1 -> Saturation/1
  Divide1/1 -> Saturation1/1
  Divide2/1 -> Saturation2/1
  [carrier] -> Relational Operator1/2
  Relational Operator1/1 -> Data Type Conversion1/1
  Saturation1/1 -> Relational Operator1/1
  [carrier] -> Relational Operator2/2
  Relational Operator2/1 -> Data Type Conversion2/1
  Data Type Conversion2/1 -> Mux/3
  Mux/1 -> q[a,b,c]/1
  Data Type Conversion/1 -> Mux/1
  Saturation/1 -> Relational Operator/1
  Data Type Conversion1/1 -> Mux/2
  Saturation2/1 -> Relational Operator2/1

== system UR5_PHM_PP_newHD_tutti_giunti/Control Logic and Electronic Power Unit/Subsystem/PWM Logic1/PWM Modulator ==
  Supply voltage : Inport
  V_ref : Inport  Port=2
  Gain1 : Gain  Gain=-1
  Product : Product  Inputs=*/
  Relational Operator : RelationalOperator  OutDataTypeStr=boolean
  Relational Operator1 : RelationalOperator  OutDataTypeStr=boolean
  Triangle Generator : spsTriangleGeneratorLib/Triangle Generator  Freq=1/T_switch  Phase=0  Ts=0
  Triangular bypolar unitary carrier : simulink/Sources/Repeating Sequence  Commented=on  rep_seq_t=[0 T_switch/4 T_switch/2 T_switch*3/4 T_switch]  rep_seq_y=[-1 0 1 0 -1]
  q1 : Outport  VectorParamsAs1DForOutWhenUnconnected=off
  q2 : Outport  Port=2  VectorParamsAs1DForOutWhenUnconnected=off
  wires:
  V_ref/1 -> Product/1
  Product/1 -> Relational Operator/1, Gain1/1
  Relational Operator/1 -> q1/1
  Gain1/1 -> Relational Operator1/1
  Triangle Generator/1 -> Relational Operator1/2, Relational Operator/2
  Relational Operator1/1 -> q2/1
  Supply voltage/1 -> Product/2

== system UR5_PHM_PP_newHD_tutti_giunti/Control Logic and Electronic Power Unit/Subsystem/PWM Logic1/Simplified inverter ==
  note: V_aO
  note: V_bO
  Supply voltage : Inport
  q1 : Inport  Port=2
  q2 : Inport  Port=3
  Product : Product  RndMeth=Zero
  Product1 : Product  RndMeth=Zero
  Sum : Sum  Inputs=|+-
  Vset : Outport  VectorParamsAs1DForOutWhenUnconnected=off
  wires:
  q1/1 -> Product/1
  q2/1 -> Product1/2
  Product/1 -> Sum/1
  Product1/1 -> Sum/2
  Sum/1 -> Vset/1
  Supply voltage/1 -> Product1/1, Product/2

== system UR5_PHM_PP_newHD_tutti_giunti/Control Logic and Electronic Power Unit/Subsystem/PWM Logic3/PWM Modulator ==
  Supply voltage : Inport
  Compensated error : Inport  Port=2
  Gain1 : Gain  Gain=-1
  Product : Product  Inputs=*/
  Relational Operator : RelationalOperator  OutDataTypeStr=boolean
  Relational Operator1 : RelationalOperator  OutDataTypeStr=boolean
  Triangle Generator : spsTriangleGeneratorLib/Triangle Generator  Freq=1/T_switch  Phase=0  Ts=0
  Triangular bypolar unitary carrier : simulink/Sources/Repeating Sequence  Commented=on  rep_seq_t=[0 T_switch/4 T_switch/2 T_switch*3/4 T_switch]  rep_seq_y=[-1 0 1 0 -1]
  q1 : Outport  VectorParamsAs1DForOutWhenUnconnected=off
  q2 : Outport  Port=2  VectorParamsAs1DForOutWhenUnconnected=off
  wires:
  Compensated error/1 -> Product/1
  Product/1 -> Relational Operator/1, Gain1/1
  Relational Operator/1 -> q1/1
  Gain1/1 -> Relational Operator1/1
  Triangle Generator/1 -> Relational Operator1/2, Relational Operator/2
  Relational Operator1/1 -> q2/1
  Supply voltage/1 -> Product/2

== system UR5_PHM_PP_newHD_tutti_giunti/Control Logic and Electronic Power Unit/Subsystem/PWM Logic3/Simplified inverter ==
  note: V_aO
  note: V_bO
  Supply voltage : Inport
  q1 : Inport  Port=2
  q2 : Inport  Port=3
  Product : Product  RndMeth=Zero
  Product1 : Product  RndMeth=Zero
  Sum : Sum  Inputs=|+-
  Vset : Outport  VectorParamsAs1DForOutWhenUnconnected=off
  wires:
  q1/1 -> Product/1
  q2/1 -> Product1/2
  Product/1 -> Sum/1
  Product1/1 -> Sum/2
  Sum/1 -> Vset/1
  Supply voltage/1 -> Product1/1, Product/2

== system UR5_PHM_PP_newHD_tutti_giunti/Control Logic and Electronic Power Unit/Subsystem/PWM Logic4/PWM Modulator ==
  Supply voltage : Inport
  Compensated error : Inport  Port=2
  Gain1 : Gain  Gain=-1
  Product : Product  Inputs=*/
  Relational Operator : RelationalOperator  OutDataTypeStr=boolean
  Relational Operator1 : RelationalOperator  OutDataTypeStr=boolean
  Triangle Generator : spsTriangleGeneratorLib/Triangle Generator  Freq=1/T_switch  Phase=0  Ts=0
  Triangular bypolar unitary carrier : simulink/Sources/Repeating Sequence  Commented=on  rep_seq_t=[0 T_switch/4 T_switch/2 T_switch*3/4 T_switch]  rep_seq_y=[-1 0 1 0 -1]
  q1 : Outport  VectorParamsAs1DForOutWhenUnconnected=off
  q2 : Outport  Port=2  VectorParamsAs1DForOutWhenUnconnected=off
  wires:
  Supply voltage/1 -> Product/2
  Relational Operator1/1 -> q2/1
  Triangle Generator/1 -> Relational Operator/2, Relational Operator1/2
  Gain1/1 -> Relational Operator1/1
  Relational Operator/1 -> q1/1
  Product/1 -> Gain1/1, Relational Operator/1
  Compensated error/1 -> Product/1

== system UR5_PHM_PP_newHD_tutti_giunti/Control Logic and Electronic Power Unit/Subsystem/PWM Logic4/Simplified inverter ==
  note: V_bO
  note: V_aO
  Supply voltage : Inport
  q1 : Inport  Port=2
  q2 : Inport  Port=3
  Product : Product  RndMeth=Zero
  Product1 : Product  RndMeth=Zero
  Sum : Sum  Inputs=|+-
  Vset : Outport  VectorParamsAs1DForOutWhenUnconnected=off
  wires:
  Supply voltage/1 -> Product/2, Product1/1
  Sum/1 -> Vset/1
  Product1/1 -> Sum/2
  Product/1 -> Sum/1
  q2/1 -> Product1/2
  q1/1 -> Product/1

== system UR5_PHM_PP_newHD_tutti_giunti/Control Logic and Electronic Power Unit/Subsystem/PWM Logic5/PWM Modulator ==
  Supply voltage : Inport
  Compensated error : Inport  Port=2
  Gain1 : Gain  Gain=-1
  Product : Product  Inputs=*/
  Relational Operator : RelationalOperator  OutDataTypeStr=boolean
  Relational Operator1 : RelationalOperator  OutDataTypeStr=boolean
  Triangle Generator : spsTriangleGeneratorLib/Triangle Generator  Freq=1/T_switch  Phase=0  Ts=0
  Triangular bypolar unitary carrier : simulink/Sources/Repeating Sequence  Commented=on  rep_seq_t=[0 T_switch/4 T_switch/2 T_switch*3/4 T_switch]  rep_seq_y=[-1 0 1 0 -1]
  q1 : Outport  VectorParamsAs1DForOutWhenUnconnected=off
  q2 : Outport  Port=2  VectorParamsAs1DForOutWhenUnconnected=off
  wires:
  Compensated error/1 -> Product/1
  Product/1 -> Relational Operator/1, Gain1/1
  Relational Operator/1 -> q1/1
  Gain1/1 -> Relational Operator1/1
  Triangle Generator/1 -> Relational Operator1/2, Relational Operator/2
  Relational Operator1/1 -> q2/1
  Supply voltage/1 -> Product/2

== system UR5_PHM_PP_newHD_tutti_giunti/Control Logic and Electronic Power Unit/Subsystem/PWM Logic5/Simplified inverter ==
  note: V_aO
  note: V_bO
  Supply voltage : Inport
  q1 : Inport  Port=2
  q2 : Inport  Port=3
  Product : Product  RndMeth=Zero
  Product1 : Product  RndMeth=Zero
  Sum : Sum  Inputs=|+-
  Vset : Outport  VectorParamsAs1DForOutWhenUnconnected=off
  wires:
  q1/1 -> Product/1
  q2/1 -> Product1/2
  Product/1 -> Sum/1
  Product1/1 -> Sum/2
  Sum/1 -> Vset/1
  Supply voltage/1 -> Product1/1, Product/2

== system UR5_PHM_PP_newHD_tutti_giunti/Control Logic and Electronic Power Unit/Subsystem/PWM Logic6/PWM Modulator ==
  Supply voltage : Inport
  Compensated error : Inport  Port=2
  Gain1 : Gain  Gain=-1
  Product : Product  Inputs=*/
  Relational Operator : RelationalOperator  OutDataTypeStr=boolean
  Relational Operator1 : RelationalOperator  OutDataTypeStr=boolean
  Triangle Generator : spsTriangleGeneratorLib/Triangle Generator  Freq=1/T_switch  Phase=0  Ts=0
  Triangular bypolar unitary carrier : simulink/Sources/Repeating Sequence  Commented=on  rep_seq_t=[0 T_switch/4 T_switch/2 T_switch*3/4 T_switch]  rep_seq_y=[-1 0 1 0 -1]
  q1 : Outport  VectorParamsAs1DForOutWhenUnconnected=off
  q2 : Outport  Port=2  VectorParamsAs1DForOutWhenUnconnected=off
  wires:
  Supply voltage/1 -> Product/2
  Relational Operator1/1 -> q2/1
  Triangle Generator/1 -> Relational Operator/2, Relational Operator1/2
  Gain1/1 -> Relational Operator1/1
  Relational Operator/1 -> q1/1
  Product/1 -> Gain1/1, Relational Operator/1
  Compensated error/1 -> Product/1

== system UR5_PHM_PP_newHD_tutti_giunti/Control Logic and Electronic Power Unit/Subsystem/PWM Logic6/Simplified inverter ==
  note: V_bO
  note: V_aO
  Supply voltage : Inport
  q1 : Inport  Port=2
  q2 : Inport  Port=3
  Product : Product  RndMeth=Zero
  Product1 : Product  RndMeth=Zero
  Sum : Sum  Inputs=|+-
  Vset : Outport  VectorParamsAs1DForOutWhenUnconnected=off
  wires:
  Supply voltage/1 -> Product/2, Product1/1
  Sum/1 -> Vset/1
  Product1/1 -> Sum/2
  Product/1 -> Sum/1
  q2/1 -> Product1/2
  q1/1 -> Product/1

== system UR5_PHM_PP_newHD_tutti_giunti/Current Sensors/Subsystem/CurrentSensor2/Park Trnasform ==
  i[a,b,c] : Inport  PortDimensions=3
  qm2 : Inport  Port=2  PortDimensions=1
  A11 : Fcn  Expr=sin(u(1))
  A12 : Fcn  Expr=cos(u(1))
  A13 : Fcn  Expr=sqrt(2)/2
  A21 : Fcn  Expr=sin(u(1)-2/3*pi)
  A22 : Fcn  Expr=cos(u(1)-2/3*pi)
  A23 : Fcn  Expr=sqrt(2)/2
  A31 : Fcn  Expr=sin(u(1)+2/3*pi)
  A32 : Fcn  Expr=cos(u(1)+2/3*pi)
  A33 : Fcn  Expr=sqrt(2)/2
  Gain : Gain  Gain=sqrt(2/3)
  Gain1 : Gain  Gain=Motor.Zp_2
  Matrix : Subsystem
  Product : Product  Multiplication=Matrix(*)  RndMeth=Zero
  i[d,q,0] : Outport  PortDimensions=[3]  InitialOutput=0  VectorParamsAs1DForOutWhenUnconnected=off
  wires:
  i[a,b,c]/1 -> Product/2
  Product/1 -> i[d,q,0]/1
  qm2/1 -> Gain1/1
  Gain/1 -> Product/1
  A21/1 -> Matrix/2(A12)
  A13/1 -> Matrix/7(A31)
  A31/1 -> Matrix/3(A13)
  A32/1 -> Matrix/6(A23)
  A11/1 -> Matrix/1(A11)
  A23/1 -> Matrix/8(A32)
  Matrix/1(Out1) -> Gain/1
  A33/1 -> Matrix/9(A33)
  A22/1 -> Matrix/5(A22)
  A12/1 -> Matrix/4(A21)
  Gain1/1 -> A12/1, A31/1, A21/1, A11/1, A33/1, A23/1, A13/1, A32/1, A22/1

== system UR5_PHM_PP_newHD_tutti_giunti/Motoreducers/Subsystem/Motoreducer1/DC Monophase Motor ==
  Vset : Inport
  C : Inport  Port=2
  Gain4 : Gain  Gain=1/Motor.Im_123
  Integrator : Integrator
  Integrator1 : Integrator  InitialCondition=q0(1)*Motor.tau
  Monophase - BLDC : Subsystem
  Mux : Mux  Inputs=3
  Sum : Sum  Inputs=|+-
  i : Outport
  qm,qdm,qddm : Outport  Port=2  VectorParamsAs1DForOutWhenUnconnected=off
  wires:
  Monophase - BLDC/2(i) -> i/1  "i_j1"
  Vset/1 -> Monophase - BLDC/1(Vset)
  Monophase - BLDC/1(T) -> Sum/1  "Tem_j1"
  Sum/1 -> Gain4/1  "Tem-C_j1"
  Gain4/1 -> Mux/3, Integrator/1
  Integrator/1 -> Monophase - BLDC/2(qdm), Mux/2, Integrator1/1
  Mux/1 -> qm,qdm,qddm/1
  Integrator1/1 -> Mux/1  "qm_j1"
  C/1 -> Sum/2  "C_j1"

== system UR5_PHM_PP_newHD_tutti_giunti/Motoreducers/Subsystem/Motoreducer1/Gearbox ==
  C : Inport
  qd : Inport  Port=2
  "  eta" : Gain  Gain=Motor.eta
  Abs : Abs
  Abs2 : Abs
  Add2 : Sum  Inputs=+|-
  Friction Function1 : Fcn  Expr=Fric1(1)*(1-tanh(Fric1(2)*u)) + Fric1(3) + Fric1(4)*u
  MinMax2 : MinMax  Inputs=2
  Product : Product  RndMeth=Zero
  Saturation : Saturate  UpperLimit=150  LowerLimit=-150
  Sign : Signum
  Sign1 : Signum
  Switch : Switch  Criteria=u2 > Threshold  Threshold=0.0
  Switch1 : Switch  Criteria=u2 > Threshold  Threshold=0.5
  Zero Detection : Fcn  Expr=abs(u(1))<1e-6
  Tu : Outport  VectorParamsAs1DForOutWhenUnconnected=off
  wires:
  qd/1 -> Zero Detection/1, Sign1/1, Abs2/1
  Switch1/1 -> Product/2
  Add2/1 -> Tu/1  "Transmitted torque [Nm]"
  Abs2/1 -> Friction Function1/1
  C/1 -> "  eta"/1
  Switch/1 -> Product/1
  MinMax2/1 -> Switch1/1
  Friction Function1/1 -> MinMax2/2, Switch1/3
  "  eta"/1 -> Saturation/1
  Product/1 -> Add2/2  "Passive torque [Nm]"
  Abs/1 -> MinMax2/1
  Zero Detection/1 -> Switch/2, Switch1/2
  Sign1/1 -> Switch/3
  Sign/1 -> Switch/1
  Saturation/1 -> Sign/1, Abs/1, Add2/1

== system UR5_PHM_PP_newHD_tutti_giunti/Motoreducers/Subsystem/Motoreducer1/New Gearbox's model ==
  Delta_q : Inport
  qm : Inport  Port=2
  Delta_qd : Inport  Port=3
  qdm : Inport  Port=4
  q : Inport  Port=5
  qd : Inport  Port=6
  Abs : Abs
  Constant1 : Constant  Value=0
  Constant2 : Constant  Value=J1.clearance
  Constant3 : Constant  Value=J1.clearance
  Mux : Mux  Inputs=3
  No Backlash : Subsystem  TreatAsAtomicUnit=on
  No contact : Subsystem  Commented=on  TreatAsAtomicUnit=on
  Scope : Scope
  "if Height < Max low altitude elseif Height > Min isotropic altitude " : If  NumInputs=4  IfExpression=u1<=1e-10  ElseIfExpressions=u2>u3, u2<u4
  phi diff > max backlash : Subsystem  Commented=on  TreatAsAtomicUnit=on
  phi diff< min backlash : Subsystem  Commented=on  TreatAsAtomicUnit=on
  C1 : Outport
  C2 : Outport  Port=2  VectorParamsAs1DForOutWhenUnconnected=off
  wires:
  Constant3/1 -> Abs/1
  [Vel_rel] -> No contact/2(In3)
  [Pos_rel] -> No contact/1(In2)
  No contact/1(Out3) -> ?
  [ELSE] -> No contact/Action
  phi diff< min backlash/1(Out1) -> ?
  phi diff > max backlash/1(Out1) -> ?
  [Pos_rel] -> phi diff< min backlash/1(In2)
  [Vel_rel] -> phi diff< min backlash/2(In3)
  [ELSEIF2] -> phi diff< min backlash/Action
  [Pos_rel] -> phi diff > max backlash/1(In2)
  [Vel_rel] -> phi diff > max backlash/2(In3)
  [IF] -> No Backlash/Action
  [ELSEIF1] -> phi diff > max backlash/Action
  "if Height < Max low altitude elseif Height > Min isotropic altitude "/3 -> [ELSEIF2]
  Constant1/1 -> Mux/3, "if Height < Max low altitude elseif Height > Min isotropic altitude "/4
  Constant2/1 -> Mux/2, "if Height < Max low altitude elseif Height > Min isotropic altitude "/3
  Abs/1 -> "if Height < Max low altitude elseif Height > Min isotropic altitude "/1
  "if Height < Max low altitude elseif Height > Min isotropic altitude "/4 -> [ELSE]
  "if Height < Max low altitude elseif Height > Min isotropic altitude "/2 -> [ELSEIF1]
  "if Height < Max low altitude elseif Height > Min isotropic altitude "/1 -> [IF]
  Delta_q/1 -> Mux/1, "if Height < Max low altitude elseif Height > Min isotropic altitude "/2, [Pos_rel]
  Mux/1 -> Scope/1
  Delta_qd/1 -> [Vel_rel]
  qm/1 -> No Backlash/1(qm)
  qdm/1 -> No Backlash/3(qdm)
  q/1 -> No Backlash/2(q)
  qd/1 -> No Backlash/4(qd)
  No Backlash/1(Ccs->giunto) -> C2/1
  No Backlash/2(Cwg->rotore) -> C1/1

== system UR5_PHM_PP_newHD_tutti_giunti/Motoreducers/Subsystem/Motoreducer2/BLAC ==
  V[ao,bo,co] : Inport
  T_w [°C] : Inport  Port=2
  C : Inport  Port=3
  Electrical dynamics-backup : Subsystem
  Electro-magnetic torque computation : Subsystem
  Integrator : Integrator
  Integrator1 : Integrator  InitialCondition=q0(2)*Motor.tau
  Motor inertia : Gain  Gain=1/Motor.Im_2
  Mux : Mux  Inputs=3
  Sum : Sum  Inputs=-+-
  Viscous Damping : Gain  Gain=Motor.ViscDamp_2
  bck-emf : Subsystem
  i[a,b,c] : Outport  VectorParamsAs1DForOutWhenUnconnected=off
  qm,qdm,qddm : Outport  Port=2
  W_joule[W] : Outport  Port=3  VectorParamsAs1DForOutWhenUnconnected=off
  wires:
  V[ao,bo,co]/1 -> Electrical dynamics-backup/1(V[ao,bo,co])
  bck-emf/2(e[a,b,c]/theta_dot) -> Electro-magnetic torque computation/2(e[a,b,c]/theta_dot)
  Electrical dynamics-backup/2(W_joule[W]) -> W_joule[W]/1
  T_w [°C]/1 -> Electrical dynamics-backup/3(T_W [*C])
  bck-emf/1(e[a,b,c]) -> Electrical dynamics-backup/2(e[a,b,c])
  Electrical dynamics-backup/1(i[a,b,c]) -> i[a,b,c]/1, Electro-magnetic torque computation/1(i[a,b,c])
  Motor inertia/1 -> Mux/3, Integrator/1  "qddm_j2"
  Integrator/1 -> Viscous Damping/1, [qdm], Mux/2, Integrator1/1  "qdm_j2"
  Integrator1/1 -> [qm], Mux/1  "qm_j2"
  Mux/1 -> qm,qdm,qddm/1
  [qm] -> bck-emf/1(qm)
  [qdm] -> bck-emf/2(qmd)
  Electro-magnetic torque computation/1(Tem) -> Sum/2  "Tem_j2"
  C/1 -> Sum/3  "C_j2"
  Sum/1 -> Motor inertia/1  "Tem-C_j2"
  Viscous Damping/1 -> Sum/1

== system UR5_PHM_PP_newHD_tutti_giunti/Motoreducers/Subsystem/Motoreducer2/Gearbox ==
  C : Inport
  qd : Inport  Port=2
  Th [°C] : Inport  Port=3
  Abs : Abs
  Abs2 : Abs
  Add2 : Sum  Inputs=+|-
  Coulomb Friction Factor : Fcn  Expr=m2(1)*u+m2(2)
  Friction Function : Fcn  Expr=Fric2(1)*(1-tanh(Fric2(2)*u)) + Fric2(3) + Fric2(4)*u
  MinMax2 : MinMax  Inputs=2
  Mux : Mux  Inputs=3
  Product : Product  RndMeth=Zero
  Saturation : Saturate  UpperLimit=150  LowerLimit=-150
  Sign : Signum
  Sign1 : Signum
  Switch : Switch  Criteria=u2 > Threshold  Threshold=0.0
  Switch1 : Switch  Criteria=u2 > Threshold  Threshold=0.5
  Viscous Friction Factor : Fcn  Expr=mb2(1)*u+mb2(2)
  Zero Detection : Fcn  Expr=abs(u(1))<1e-6
  eta : Gain  Gain=Motor.eta
  Tu : Outport  VectorParamsAs1DForOutWhenUnconnected=off
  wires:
  eta/1 -> Saturation/1
  Switch/1 -> Product/1
  MinMax2/1 -> Switch1/1
  Add2/1 -> Tu/1  "Transmitted torque [Nm]"
  C/1 -> eta/1
  Sign/1 -> Switch/1
  Abs/1 -> MinMax2/1
  Friction Function/1 -> MinMax2/2, Switch1/3
  Product/1 -> Add2/2  "Passive torque [Nm]"
  Switch1/1 -> Product/2
  Zero Detection/1 -> Switch/2, Switch1/2
  Sign1/1 -> Switch/3
  qd/1 -> Abs2/1, Zero Detection/1, Sign1/1
  Abs2/1 -> Mux/1
  Viscous Friction Factor/1 -> Mux/3
  Coulomb Friction Factor/1 -> Mux/2
  Th [°C]/1 -> Viscous Friction Factor/1, Coulomb Friction Factor/1
  Mux/1 -> Friction Function/1
  Saturation/1 -> Abs/1, Sign/1, Add2/1

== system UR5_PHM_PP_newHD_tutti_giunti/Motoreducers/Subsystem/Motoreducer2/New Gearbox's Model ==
  Delta_q : Inport
  qm : Inport  Port=2
  Delta_qd : Inport  Port=3
  qdm : Inport  Port=4
  q : Inport  Port=5
  qd : Inport  Port=6
  Abs : Abs
  Constant1 : Constant  Value=0
  Constant2 : Constant  Value=J2.clearance
  Constant3 : Constant  Value=J2.clearance
  Mux : Mux  Inputs=3
  No Backlash : Subsystem  TreatAsAtomicUnit=on
  No contact : Subsystem  Commented=on  TreatAsAtomicUnit=on
  Scope : Scope
  "if Height < Max low altitude elseif Height > Min isotropic altitude " : If  NumInputs=4  IfExpression=u1<=1e-10  ElseIfExpressions=u2>u3, u2<u4
  phi diff > max backlash : Subsystem  Commented=on  TreatAsAtomicUnit=on
  phi diff< min backlash : Subsystem  Commented=on  TreatAsAtomicUnit=on
  C1 : Outport
  C2 : Outport  Port=2  VectorParamsAs1DForOutWhenUnconnected=off
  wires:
  "if Height < Max low altitude elseif Height > Min isotropic altitude "/4 -> [ELSE]
  No contact/1(Out3) -> ?
  "if Height < Max low altitude elseif Height > Min isotropic altitude "/1 -> [IF]
  Constant3/1 -> Abs/1
  "if Height < Max low altitude elseif Height > Min isotropic altitude "/2 -> [ELSEIF1]
  Delta_qd/1 -> [Vel_rel]
  [Vel_rel] -> phi diff< min backlash/2(In3)
  [Vel_rel] -> No contact/2(In3)
  Mux/1 -> Scope/1
  Constant2/1 -> Mux/2, "if Height < Max low altitude elseif Height > Min isotropic altitude "/3  "clearance_j2"
  Delta_q/1 -> "if Height < Max low altitude elseif Height > Min isotropic altitude "/2, Mux/1, [Pos_rel]
  Constant1/1 -> Mux/3, "if Height < Max low altitude elseif Height > Min isotropic altitude "/4
  [Vel_rel] -> phi diff > max backlash/2(In3)
  phi diff< min backlash/1(Out1) -> ?
  [ELSEIF1] -> phi diff > max backlash/Action
  [IF] -> No Backlash/Action
  [Pos_rel] -> phi diff > max backlash/1(In2)
  [ELSEIF2] -> phi diff< min backlash/Action
  No Backlash/1(Ccs->giunto) -> C2/1  "C [Nm]"
  phi diff > max backlash/1(Out1) -> ?
  "if Height < Max low altitude elseif Height > Min isotropic altitude "/3 -> [ELSEIF2]
  Abs/1 -> "if Height < Max low altitude elseif Height > Min isotropic altitude "/1
  [Pos_rel] -> No contact/1(In2)
  [ELSE] -> No contact/Action
  [Pos_rel] -> phi diff< min backlash/1(In2)
  qm/1 -> No Backlash/1(qm)
  q/1 -> No Backlash/2(q)
  qdm/1 -> No Backlash/3(qdm)
  qd/1 -> No Backlash/4(qd)
  No Backlash/2(Cwg->rotore) -> C1/1
